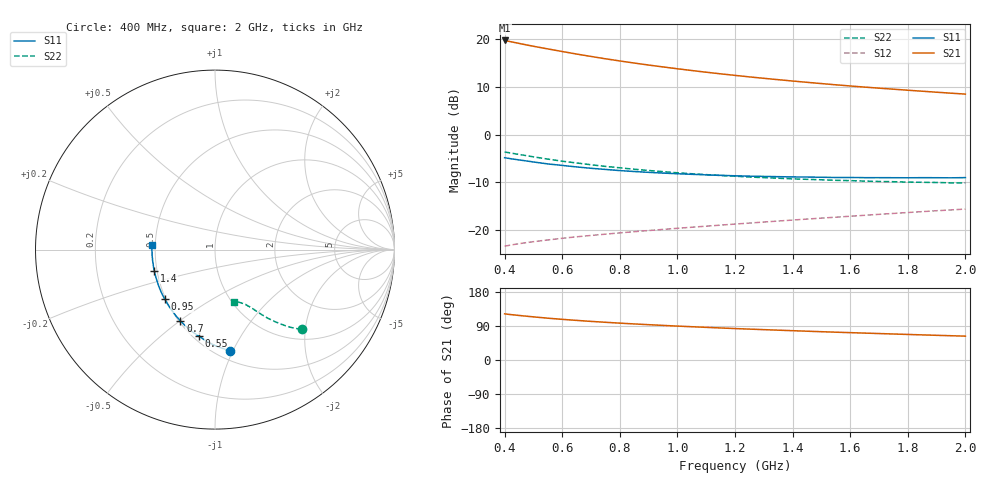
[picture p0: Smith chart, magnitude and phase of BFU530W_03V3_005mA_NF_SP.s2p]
! Filename:  P:\Prog\Test\Noise\ATS_data\Testdata_Net\06 Compressed Noise after Statistics\BFU530W_APM2013_09_A05_03p3V_005mA_NF_CM01_D.sf
! Date/Time: Tue 26/Mar/2013 18:06:07
! BFU530W_APM2013_09_A05_03p3V_1to25mA_NF_CM01_Bias4_R.sf
! Noise Parameter Data File
! BFU530W_APM2013_09_A05_03p3V_1to25mA_NF_CM01
! Date/time: Thu Mar 21 19:18:02 2013
! VAR V_out= 3.300000
! VAR I_out= 5.000000
! VAR V_in= 0.821800
! VAR I_in= 0.053210
! Device data file deembeded for feedlines and parallel
! Original file: \06 Compressed Noise after Statistics\BFU530W_APM2013_09_A05_03p3V_005mA_NF_CM01_R.sf
! Feed-files: PR019V01_070313_Feed1.s2p, PR019V01_070313_Feed2.s2p
! Parallel-file: PR019V01_070313_Par.s2p
# MHz S MA R 50
!  Freq-MHz  S11-mag  S11-arg  S21-mag  S21-arg  S12-mag  S12-arg  S22-mag  S22-arg
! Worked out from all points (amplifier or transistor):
!   37 points, 400 MHz to 2 GHz, reference 50 ohm
!   highest |S21| = 19.8 dB at 400 MHz (marker M1)
!   |S21| within 3 dB of that: start of sweep to 663.6 MHz
!   unconditionally stable (mu >= 1): 1.768 GHz to end of sweep
!   at 500 MHz: K = 0.51, MSG = 20.6 dB, |S12| = -22.5 dB
!   at 1.1 GHz: K = 0.86, MSG = 16.2 dB, |S12| = -19.3 dB
!   at 2 GHz: K = 1.02, MAG = 11.3 dB, |S12| = -15.7 dB
!   lowest NFmin = 0.59 dB at 420 MHz
!   S11 on the Smith chart (normalised r, x): 400 MHz: 0.58, -0.98; 550 MHz: 0.53, -0.68; 700 MHz: 0.51, -0.50; 950 MHz: 0.49, -0.32; 1.4 GHz: 0.48, -0.13; 2 GHz: 0.48, +0.03
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400  0.5702 -81.4  9.769 121.7  0.06692 55.8  0.6557 -42.6
420  0.5576 -84.3  9.496 120.0  0.06864 55.2  0.6399 -43.6
440  0.5463 -87.0  9.23 118.3  0.07023 54.6  0.6246 -44.5
480  0.5253 -92.2  8.722 115.3  0.07322 53.7  0.5966 -46.2
500  0.5146 -94.8  8.488 113.8  0.07459 53.3  0.5826 -47.0
550  0.4909 -100.5  7.96 110.4  0.07778 52.7  0.5516 -48.6
600  0.4733 -106.1  7.477 107.3  0.081 52.2  0.5245 -50.1
650  0.4563 -111.0  7.025 104.5  0.08397 51.9  0.5022 -51.3
700  0.4415 -115.8  6.631 101.9  0.08676 51.7  0.4812 -52.5
750  0.4294 -120.2  6.268 99.5  0.08952 51.7  0.4622 -53.4
800  0.4175 -124.3  5.946 97.3  0.09232 51.8  0.4469 -54.3
850  0.4083 -128.4  5.652 95.2  0.09503 51.9  0.4314 -55.0
950  0.393 -135.4  5.145 91.3  0.1004 52.4  0.4072 -56.5
1050  0.3815 -142.0  4.715 87.8  0.1058 52.9  0.3869 -57.7
1150  0.3722 -148.1  4.35 84.5  0.1114 53.4  0.3706 -59.0
1200  0.3681 -150.8  4.192 83.0  0.1143 53.7  0.3645 -59.6
1300  0.3625 -156.1  3.904 80.1  0.12 54.3  0.3518 -60.7
1400  0.3583 -161.0  3.656 77.3  0.126 54.9  0.3416 -61.9
1500  0.3551 -165.4  3.437 74.7  0.132 55.3  0.3344 -63.4
1600  0.3532 -169.8  3.244 72.2  0.1382 55.8  0.3275 -64.5
1750  0.3514 -175.5  3 68.6  0.1479 56.3  0.319 -66.5
2000  0.3523 175.5  2.664 63.0  0.1645 56.9  0.3097 -70.2
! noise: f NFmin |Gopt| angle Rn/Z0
400  0.5953  0.1652  39.66  0.1026
460  0.591  0.1691  43.84  0.102
600  0.6209  0.1764  49.67  0.1037
800  0.6857  0.1725  69.68  0.0943
1000  0.7005  0.1797  84.54  0.0947
1200  0.756  0.1928  99.37  0.0892
1400  0.7611  0.212  113.9  0.0835
1600  0.752  0.2223  129.9  0.0758
1800  0.8326  0.2536  145.8  0.0649
2000  0.8649  0.3037  156.4  0.0572
